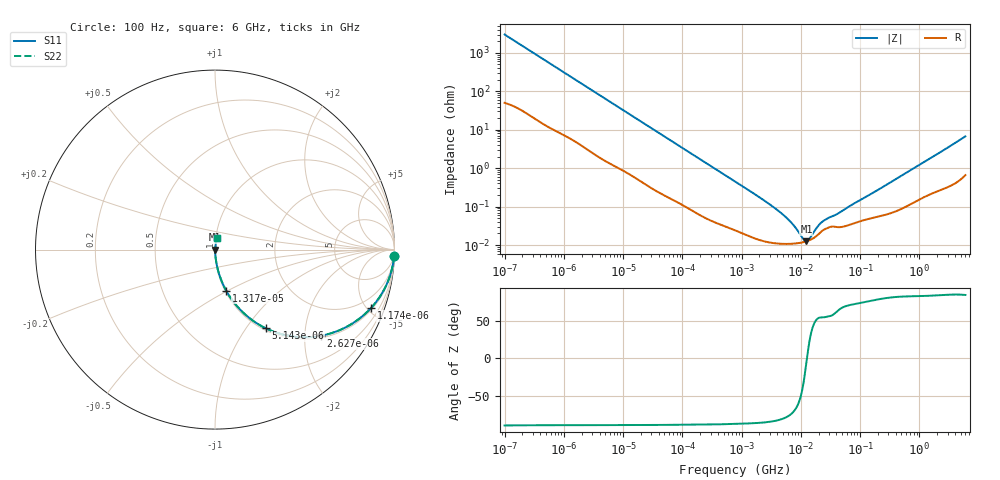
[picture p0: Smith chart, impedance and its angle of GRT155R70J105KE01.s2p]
!Murata Part Number: GRT155R70J105KE01
!These Parameters are Measured in Series Mode Connection
!Data Generated on Jun 19, 2026
!  o--ll--o
!Port1  Port2
!  o------o
!Operation Temp=25[degC], DC Bias Voltage=0[V]
!Freq. Start=100[Hz] Stop=6[GHz] 401[Steps]
# Hz S RI R 50
!Freq.(Hz) S11(Real) S11(Imag) S21(Real) S21(Imag) S12(Real) S12(Imag) S22(Real) S22(Imag)
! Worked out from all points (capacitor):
!   401 points, 100 Hz to 6 GHz, reference 50 ohm
!   read as one part in series: C = 526 nF near 109 Hz
!   lowest |Z| = 12.5 mohm at 12.44 MHz (marker M1)
!   series resonance near 12.69 MHz, so ESL is about 300 pH
!   S11 on the Smith chart (normalised r, x): 100 Hz: 2, -60; 1.174 kHz: 1.13, -5.31; 2.627 kHz: 1.06, -2.41; 5.143 kHz: 1.03, -1.24; 13.17 kHz: 1.01, -0.49; 6 GHz: 1.01, +0.13
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100  0.9983 -0.0331  0.00165 0.0331  0.00165 0.0331  0.9983 -0.0331
401  0.9808 -0.1275  0.0192 0.1275  0.0192 0.1275  0.9808 -0.1275
1174  0.8701 -0.3245  0.1299 0.3245  0.1299 0.3245  0.8701 -0.3245
2008  0.7061 -0.4435  0.2939 0.4435  0.2939 0.4435  0.7061 -0.4435
2627  0.5893 -0.4801  0.4107 0.4801  0.4107 0.4801  0.5893 -0.4801
5143  0.2825 -0.4383  0.7175 0.4383  0.7175 0.4383  0.2825 -0.4383
8047  0.1437 -0.3381  0.8563 0.3381  0.8563 0.3381  0.1437 -0.3381
13169  0.0626 -0.229  0.9374 0.229  0.9374 0.229  0.0626 -0.229
40335  0.00891 -0.0809  0.9911 0.0809  0.9911 0.0809  0.00891 -0.0809
774597  0.000261 -0.0045  0.9997 0.0045  0.9997 0.0045  0.000261 -0.0045
2372521  0.000128 -0.00146  0.9999 0.00146  0.9999 0.00146  0.000128 -0.00146
4643984  0.000108 -0.000672  0.9999 0.000672  0.9999 0.000672  0.000108 -0.000672
7266822  0.000108 -0.000334  0.9999 0.000334  0.9999 0.000334  0.000108 -0.000334
1.087309e7  0.000118 -8.84e-05  0.9999 8.84e-05  0.9999 8.84e-05  0.000118 -8.84e-05
1.243624e7  0.000125 -1.13e-05  0.9999 1.13e-05  0.9999 1.13e-05  0.000125 -1.13e-05
1.360128e7  0.000131 4e-05  0.9999 -4e-05  0.9999 -4e-05  0.000131 4e-05
1.555665e7  0.000144 0.000118  0.9999 -0.000118  0.9999 -0.000118  0.000144 0.000118
1.946e7  0.000185 0.000248  0.9998 -0.000248  0.9998 -0.000248  0.000185 0.000248
2.434276e7  0.000249 0.000349  0.9998 -0.000349  0.9998 -0.000349  0.000249 0.000349
4.165952e7  0.000293 0.000577  0.9997 -0.000577  0.9997 -0.000577  0.000293 0.000577
3.124326e8  0.000671 0.00404  0.9993 -0.00404  0.9993 -0.00404  0.000671 0.00404
6e9  0.0109 0.0658  0.9891 -0.0658  0.9891 -0.0658  0.0109 0.0658
